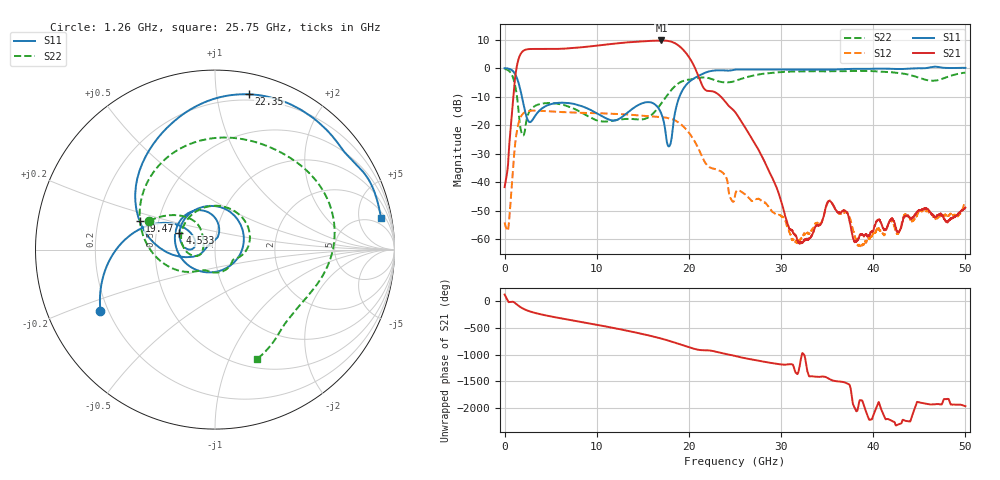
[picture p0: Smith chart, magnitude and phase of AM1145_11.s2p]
!Agilent Technologies,E8364B,MY43040894,A.07.50.67
!Agilent E8364B: A.07.50.67
!Date: Monday, November 15, 2021 11:32:15
!Correction: S11(Full 2 Port(1,2))
!S21(Full 2 Port(1,2))
!S12(Full 2 Port(1,2))
!S22(Full 2 Port(1,2))
!S2P File: Measurements: S11, S21, S12, S22:
# Hz S  dB  R 50
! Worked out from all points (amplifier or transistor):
!   6401 points, 10 MHz to 50 GHz, reference 50 ohm
!   highest |S21| = 9.7 dB at 17.02 GHz (marker M1)
!   |S21| within 3 dB of that: 5.291 GHz to 19.31 GHz (14.02 GHz wide, 114 % of centre)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
!   unconditionally stable (mu >= 1): start of sweep to 45.77 GHz
!   at 8.336 GHz: K = 1.41, MAG = 7.7 dB, |S12| = -15.7 dB
!   at 25 GHz: K = 38.96, MAG = -4.2 dB, |S12| = -44.7 dB
!   at 50 GHz: K = -150.59, MSG = -1.1 dB, |S12| = -46.7 dB
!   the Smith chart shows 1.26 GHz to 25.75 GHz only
!   S11 on the Smith chart (normalised r, x): 1.26 GHz: 0.17, -0.24; 4.533 GHz: 0.66, +0.13; 19.47 GHz: 0.39, +0.16; 22.35 GHz: 0.15, +1.23; 25.75 GHz: 3, +10
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1e7  -0.05 -12.4  -41.70 130.9  -54.03 65.0  -0.25 -16.8
1.25975e9  -2.81 -151.9  -0.78 -44.8  -23.80 169.6  -7.97 156.4
1.822138e9  -9.06 155.5  5.31 -115.8  -16.75 91.6  -22.45 147.9
2.59542e9  -18.58 158.7  6.63 -177.9  -15.02 24.0  -15.90 -176.3
4.532533e9  -13.21 154.9  6.66 95.7  -15.07 -66.3  -12.27 94.9
6.59462e9  -12.16 102.3  6.84 27.8  -15.46 -133.0  -13.08 33.1
8.34427e9  -13.30 58.9  7.28 -26.5  -15.66 175.9  -15.54 -5.0
1.07969e10  -17.22 -16.9  8.15 -104.5  -15.87 105.0  -18.75 -30.8
1.313238e10  -16.15 -134.7  8.94 175.5  -16.20 34.8  -17.81 -69.7
1.512416e10  -12.13 148.6  9.38 101.2  -16.72 -28.1  -17.88 -114.9
1.667854e10  -13.92 96.6  9.66 36.5  -17.08 -81.9  -13.82 -142.5
1.702222e10  -16.02 85.4  9.67 20.7  -17.17 -95.1  -12.34 -151.9
1.844381e10  -16.51 -163.8  8.79 -53.4  -18.24 -157.7  -6.48 152.1
1.946705e10  -6.93 159.0  6.13 -111.6  -20.66 151.8  -4.41 104.9
2.076366e10  -3.22 118.6  -0.69 179.8  -26.43 89.6  -3.67 54.8
2.234928e10  -1.05 77.6  -8.04 155.1  -34.87 56.4  -3.71 -1.8
2.5005e10  -0.56 25.7  -15.33 53.5  -44.66 16.6  -4.51 -54.4
2.575485e10  -0.52 10.8  -19.00 23.6  -43.46 -36.0  -3.70 -68.9
3.333927e10  -0.54 -110.5  -58.46 29.0  -56.66 58.0  -1.07 160.6
4.167354e10  -0.23 158.2  -54.26 -58.5  -54.28 -49.0  -1.37 66.6
4.660224e10  0.50 126.8  -52.05 -139.5  -52.37 -26.2  -4.43 -86.5
5e10  0.07 104.6  -48.86 -173.6  -46.65 -152.0  -1.60 151.5
